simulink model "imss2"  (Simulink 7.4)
settings: Solver=ode45  StartTime=0.0  StopTime=0  MaxStep=3
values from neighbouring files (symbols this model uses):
  Lm = eval(get(hLm,'String'))    [im3d.m]    (also in IMabc2.m = 4.5; imabcparam.m = 0.0847; IMabcrun0.m = 0.0847; IMabcrun1.m = 0.0847)
  Lrl = eval(get(hLr,'String'))    [im3d.m]    (also in IMabc2.m = 0.1; imabcparam.m = 0.0025; IMabcrun0.m = 0.0025; IMabcrun1.m = 0.0025)
  Lsl = eval(get(hLs,'String'))    [im3d.m]    (also in IMabc2.m = 0.1; imabcparam.m = 0.0025; IMabcrun0.m = 0.0025; IMabcrun1.m = 0.0025)
  Rr = input('Rotor resistance)[default = 2] =')    [Actac.m]    (also in im1phase.m = 0.3; im3d.m = eval(get(hRr,'String')); IMabc2.m = 0.02; imabcparam.m = 0.408)
  Rs = eval(get(hRs,'String'))    [im3d.m]    (also in IMabc2.m = 0.01; imabcparam.m = 0.531; IMabcrun0.m = 0.531; IMabcrun1.m = 0.531)
  V = [Vas 0 0].'    [Actac.m]    (also in acttrcalc1.m = str2num(get(h,'string')); im3d.m = eval(get(hVs,'String')); IMabc2.m = [vas vbs vcs 0 0 0]'; IMabcf0.m = [vas vbs vcs 0 0 0]')
  wm = x(7)    [IMabc2.m]    (also in IMabcf0.m; IMabcf1.m; IMcurf0.m = x(5))
  ws = 1.0    (= 1)    [IMabc2.m]    (also in IMcur0.m; imdef0vec.m; imdef1vec.m; imdef2vec.m)

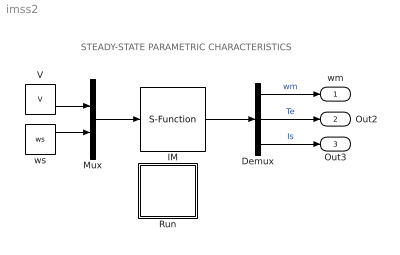
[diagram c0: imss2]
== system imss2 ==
  note: STEADY-STATE PARAMETRIC CHARACTERISTICS
  Demux : Demux  Outputs=3
  IM : S-Function  FunctionName=imssmod2  Parameters=Rs,Rr,Lsl,Lrl,Lm,wm  EnableBusSupport=off
  Mux : Mux  Inputs=2
  Run : Subsystem
  V : Constant  Value=V  OutDataType=sfix(16)  OutScaling=2^0
  ws : Constant  Value=ws  OutDataType=sfix(16)  OutScaling=2^0
  wm : Outport
  Out2 : Outport  Port=2
  Out3 : Outport  Port=3
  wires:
  ws/1 -> Mux/2
  V/1 -> Mux/1
  Mux/1 -> IM/1
  IM/1 -> Demux/1
  Demux/3 -> Out3/1  "Is"
  Demux/1 -> wm/1  "wm"
  Demux/2 -> Out2/1  "Te"

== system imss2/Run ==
  note: This demo illustrates the steady-state characteristics of an induction motor in the form of torque-speed and current-speed curves
  note: Double click
  note: Edit to modify the parameters
